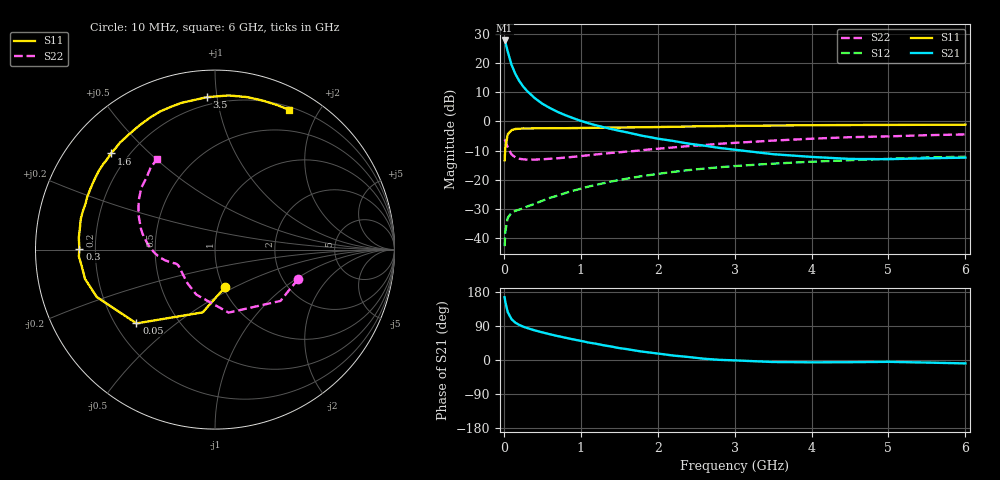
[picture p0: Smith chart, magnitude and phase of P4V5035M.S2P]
! SIEMENS Small Signal Semiconductors
! BFP182
! Si NPN RF Bipolar Junction Transistor in SOT143
! VCE = 0.5 V  IC = 35 mA
! Common Emitter S-Parameters:  March  1996
# GHz  S  MA  R  50
!  f  S11  S21  S12  S22
! GHz  MAG  ANG  MAG  ANG  MAG  ANG  MAG  ANG
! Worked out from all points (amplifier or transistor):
!   36 points, 10 MHz to 6 GHz, reference 50 ohm
!   highest |S21| = 27.8 dB at 10 MHz (marker M1)
!   |S21| within 3 dB of that: start of sweep to 42.78 MHz
!   unconditionally stable (mu >= 1): start of sweep to 29.09 MHz; 120.9 MHz to end of sweep
!   at 250 MHz: K = 1.61, MAG = 16.4 dB, |S12| = -29.9 dB
!   at 1.4 GHz: K = 2.67, MAG = 1.9 dB, |S12| = -20.6 dB
!   at 6 GHz: K = 1.74, MAG = -5.2 dB, |S12| = -12.1 dB
!   S11 on the Smith chart (normalised r, x): 10 MHz: 1.02, -0.45; 50 MHz: 0.29, -0.37; 300 MHz: 0.14, +0.00; 1.6 GHz: 0.14, +0.38; 3.5 GHz: 0.15, +0.94; 6 GHz: 0.23, +1.64
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0.01  0.2157 -74.5  24.64 165.8  0.0072 64.6  0.4911 -19.6
0.02  0.3564 -101.1  22.97 152.9  0.013 60.3  0.4634 -38.1
0.05  0.6004 -136.8  15.99 126.7  0.022 43.7  0.3592 -77.8
0.1  0.7095 -158.1  9.403 107.6  0.0271 31.7  0.2715 -112.5
0.15  0.7424 -167.3  6.558 98.5  0.0292 30.7  0.2418 -129.6
0.2  0.7488 -173.2  4.971 92.6  0.0306 32.9  0.2285 -139.4
0.25  0.7594 -177.1  4.007 88.1  0.0321 34.1  0.2239 -145.9
0.3  0.7559 179.7  3.362 84.5  0.0345 37.3  0.2211 -149.9
0.4  0.7617 174.9  2.531 78.3  0.0384 41.8  0.2212 -154.6
0.5  0.7625 170.7  2.018 72.9  0.0434 44.2  0.2238 -157.6
0.6  0.7672 167.1  1.698 67.8  0.0487 47.2  0.2286 -159.6
0.7  0.7667 163.7  1.459 63.2  0.0532 49.2  0.2334 -160.5
0.8  0.7654 160.5  1.28 58.8  0.0589 50.2  0.2395 -161.5
1.1  0.7751 151.3  0.933 46.1  0.0761 51.0  0.2632 -164.8
1.3  0.7821 145.8  0.796 38.7  0.0871 50.4  0.2797 -167.3
1.6  0.7897 137.3  0.65 28.7  0.1041 48.4  0.3043 -171.0
2.2  0.8097 121.5  0.463 11.8  0.1359 42.0  0.3575 179.0
2.8  0.8327 107.0  0.351 0.4  0.1634 34.2  0.4128 167.8
3.5  0.8505 93.0  0.274 -5.3  0.1884 25.3  0.4692 155.4
4.5  0.8686 77.9  0.227 -5.8  0.2158 13.7  0.5367 139.8
5.5  0.8763 66.9  0.233 -6.8  0.2406 3.5  0.581 128.1
6  0.8817 62.0  0.239 -9.0  0.2479 -2.1  0.5992 122.4
